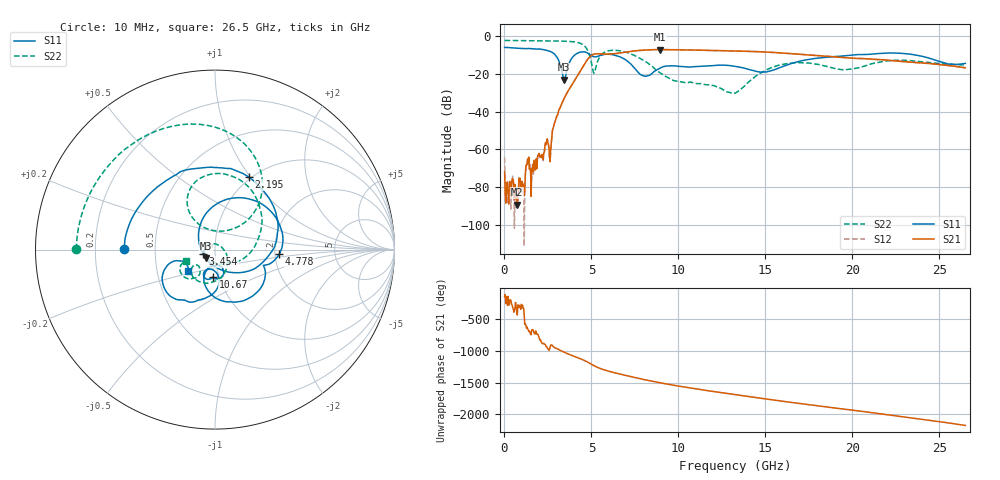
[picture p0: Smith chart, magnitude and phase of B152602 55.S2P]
!  2-Port S-parameters saved by WinCal
! VAR MeasName=S-Parameters (CALIBRATED_DATA) read from VNA (N5242A)
! VAR MeasDate=2016-1-5 16:33:51
! VAR NAME=B152602 55
! VAR FILENAME=B152602 55.S2P
! VAR DATE=2016-1-5 16:33:51
! VAR PHYS_PORTS=1,2
# Hz S DB R 50
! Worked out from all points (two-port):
!   801 points, 10 MHz to 26.5 GHz, reference 50 ohm
!   highest |S21| = -7.07 dB at 8.95 GHz (marker M1); lowest = -89.3 dB at 738.5 MHz (marker M2)
!   |S21| within 3 dB of the highest: 5.02 GHz to 17.71 GHz (12.69 GHz wide, 112 % of centre)
!   lowest |S11| = -23.1 dB at 3.421 GHz (marker M3), VSWR 1.15, Z = 45 - j4.43 ohm
!   |S11| at or under -10 dB: 2.928 GHz to 4.035 GHz (1.108 GHz wide, 31.8 % of centre); 6.324 GHz to 19.94 GHz (13.61 GHz wide, 104 % of centre); 23.66 GHz to end of sweep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
!   |S22| runs from -30.3 to -2.2 dB; largest |S21 - S12| = 0.0032
!   S11 on the Smith chart (normalised r, x): 10 MHz: 0.33, +0.00; 2.195 GHz: 0.97, +0.98; 3.454 GHz: 0.88, -0.04; 4.778 GHz: 2.11, -0.12; 10.67 GHz: 0.94, -0.29; 26.5 GHz: 0.72, -0.18
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1e7  -5.93 179.4  -71.96 -134.6  -64.35 -96.1  -2.24 179.9
1.755625e8  -5.97 170.9  -82.13 80.9  -76.80 82.0  -2.24 177.3
7.38475e8  -6.35 143.8  -89.29 -67.8  -87.58 90.4  -2.28 168.6
1.367612e9  -6.46 114.1  -67.37 57.4  -65.86 62.0  -2.33 158.7
2.195425e9  -7.01 65.2  -64.40 -158.9  -65.15 -164.7  -2.41 144.8
2.625888e9  -8.02 31.6  -66.56 142.2  -65.23 138.5  -2.45 136.7
3.420588e9  -23.06 -135.8  -33.25 64.6  -33.25 64.7  -2.62 118.5
3.4537e9  -23.04 -159.5  -32.56 60.2  -32.57 60.1  -2.63 117.6
4.447075e9  -8.31 24.6  -17.13 -50.1  -17.13 -50.0  -4.09 76.8
4.7782e9  -8.90 -4.1  -12.31 -93.4  -12.31 -93.3  -7.42 51.7
5.17555e9  -10.95 -17.8  -9.43 -154.7  -9.42 -154.6  -19.31 97.7
5.70535e9  -9.72 -34.0  -9.48 145.1  -9.47 145.2  -8.74 112.3
6.6325e9  -10.87 -82.8  -8.89 76.9  -8.88 76.9  -7.69 70.3
7.990112e9  -21.06 -94.2  -7.40 -8.8  -7.39 -8.7  -12.73 8.2
8.851038e9  -17.40 -69.1  -7.08 -56.6  -7.06 -56.6  -18.83 -39.9
8.950375e9  -16.90 -70.4  -7.07 -61.9  -7.06 -62.0  -19.45 -46.6
1.067222e10  -16.35 -93.8  -7.28 -143.3  -7.26 -143.3  -24.25 -166.8
1.3255e10  -15.97 -113.1  -7.84 111.3  -7.82 111.2  -30.18 53.9
1.553976e10  -17.69 -85.9  -8.63 23.4  -8.61 23.3  -16.02 -77.9
1.769208e10  -11.99 -93.9  -10.06 -55.1  -10.01 -54.9  -14.49 -133.2
2.209604e10  -8.87 -134.4  -12.79 150.2  -12.72 149.9  -12.97 -134.6
2.65e10  -14.36 -141.9  -16.75 -17.0  -16.75 -17.0  -15.27 -157.8
